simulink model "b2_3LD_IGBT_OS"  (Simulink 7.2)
settings: Solver=ode3  SolverMode=SingleTasking  StartTime=0.0  StopTime=0.2  FixedStep=10e-6  MaxStep=1e-5  RelTol=1e-4  AbsTol=1e-4

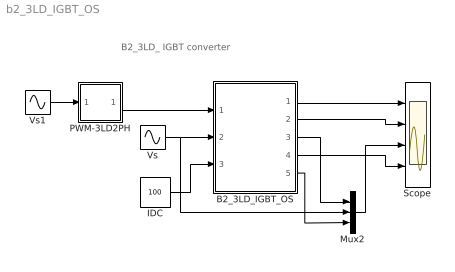
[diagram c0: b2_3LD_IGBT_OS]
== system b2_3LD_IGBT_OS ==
  note: B2_3LD_ IGBT converter
  B2_3LD_IGBT_OS : Subsystem  mask(B2-3-Level NPC IGBT Converter){LS=2e-3, C=20e-3, VC0=200, RL=10e5}
      mask prompts: LS "Source Inductance"; C "Load Cap"; VC0 "Initial Cap Voltage"; RL "Load Resistance"
      mask help: Input Vector u: u[0]= IGBT1.gate u[1]= IGBT2.gate u[2]= IGBT3.gate u[3]= IGBT4.gate u[4]= IGBT5.gate u[5]= IGBT6.gate u[6]= IGBT7.gate u[7]= IGBT8.gate u[8]= V1.V u[9]= IDC.i Output Vector y: y[0]= T1.I y[1]= D1.I y[2]= T1.V y[3]= T2.I y[4]= D2.I y[5]= T2.V y[6]= LS1.I y[7]= DC.V y[8]= Va.V Parameter Vector p: p[0]= Ls.L p[1]= C1.C p[2]= C1.vC0 p[3]= R1.r You can pause the simulation during running, change the Parameters you want and continue the Simulation
  IDC : Constant  Value=100
  Mux2 : Mux  Inputs=3
  PWM-3LD2PH : Subsystem  mask(PWM-3LD_3PH){FT=900, PHT=0, A=0.5, O1=0.5, O2=-0.5, DT=1e-6}
      mask prompts: FT "Frequency of Trian Sig."; PHT "Phase Angle of Trian. Sig."; A "Amplitude of Trian. Sig."; O1 "Offset of 1st Trian"; O2 "Offset of 2nd Trian."; DT "Dead Time"
      mask help: Pulse Width Modulation for 2 Legs of 3 Level Neutral point clamped Converter
  Scope : Scope  NumInputPorts=4
  Vs : Sin  Amplitude=230*sqrt(2)  Frequency=50*2*pi  SampleTime=0
  Vs1 : Sin  Amplitude=0.74  Frequency=50*2*pi  Phase=-pi/6  SampleTime=0
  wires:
  IDC/1 -> B2_3LD_IGBT_OS/3(iDC)
  B2_3LD_IGBT_OS/1(iT1,iD1,vT1) -> Scope/1
  B2_3LD_IGBT_OS/2(iT2,iD2,vT2) -> Scope/2
  B2_3LD_IGBT_OS/4(vDC12) -> Scope/4
  Vs/1 -> Mux2/2, B2_3LD_IGBT_OS/2(vS)
  Vs1/1 -> PWM-3LD2PH/1(In1)
  B2_3LD_IGBT_OS/3(iLs) -> Mux2/1
  Mux2/1 -> Scope/3
  B2_3LD_IGBT_OS/5(va) -> Mux2/3
  PWM-3LD2PH/1(Out1) -> B2_3LD_IGBT_OS/1(SWs)

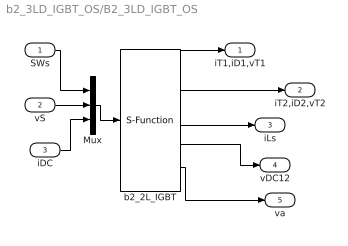
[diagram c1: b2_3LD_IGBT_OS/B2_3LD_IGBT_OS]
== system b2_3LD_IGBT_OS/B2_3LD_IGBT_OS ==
  SWs : Inport  OutDataType=sfix(16)  OutScaling=2^0
  vS : Inport  Port=2  OutDataType=sfix(16)  OutScaling=2^0
  iDC : Inport  Port=3  OutDataType=sfix(16)  OutScaling=2^0
  Mux : Mux  Inputs="[8  1  1]"
  b2_2L_IGBT : S-Function  FunctionName=s_b2_3LD_IGBT_OS  Parameters="[ LS  C  VC0 RL]"  EnableBusSupport=off
  iT1,iD1,vT1 : Outport  OutDataType=sfix(16)  OutScaling=2^0
  iT2,iD2,vT2 : Outport  Port=2  OutDataType=sfix(16)  OutScaling=2^0
  iLs : Outport  Port=3  OutDataType=sfix(16)  OutScaling=2^0
  vDC12 : Outport  Port=4  OutDataType=sfix(16)  OutScaling=2^0
  va : Outport  Port=5  OutDataType=sfix(16)  OutScaling=2^0
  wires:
  b2_2L_IGBT/4 -> vDC12/1
  Mux/1 -> b2_2L_IGBT/1
  iDC/1 -> Mux/3
  b2_2L_IGBT/3 -> iLs/1
  b2_2L_IGBT/2 -> iT2,iD2,vT2/1
  b2_2L_IGBT/1 -> iT1,iD1,vT1/1
  vS/1 -> Mux/2
  SWs/1 -> Mux/1
  b2_2L_IGBT/5 -> va/1

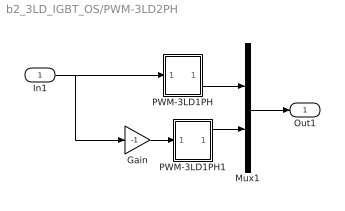
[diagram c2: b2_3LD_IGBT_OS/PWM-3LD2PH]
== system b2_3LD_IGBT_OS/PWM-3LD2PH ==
  In1 : Inport  OutDataType=sfix(16)  OutScaling=2^0
  Gain : Gain  Gain=-1  ParameterDataType=sfix(16)  ParameterScaling=2^0  OutDataType=sfix(16)  OutScaling=2^0
  Mux1 : Mux  Inputs=2
  PWM-3LD1PH : Subsystem  mask(PWM-3LD1PH){FT=FT, PHT=PHT, A=A, O1=O1, O2=O2, DT=DT}
      mask prompts: FT "Frequency of Trian Sig."; PHT "Phase Angle of Trian. Sig."; A "Amplitude of Trian. Sig."; O1 "Offset of 1st Trian"; O2 "Offset of 2nd Trian."; DT "Dead Time"
      mask help: Pulse Width Modulation for 1 Phase 3 Level Floating Capacitor Converter
  PWM-3LD1PH1 : Subsystem  mask(PWM-3LD1PH){FT=FT, PHT=PHT, A=A, O1=O1, O2=O2, DT=DT}
      mask prompts: FT "Frequency of Trian Sig."; PHT "Phase Angle of Trian. Sig."; A "Amplitude of Trian. Sig."; O1 "Offset of 1st Trian"; O2 "Offset of 2nd Trian."; DT "Dead Time"
      mask help: Pulse Width Modulation for 1 Phase 3 Level Floating Capacitor Converter
  Out1 : Outport
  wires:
  PWM-3LD1PH1/1(Out1) -> Mux1/2
  PWM-3LD1PH/1(Out1) -> Mux1/1
  In1/1 -> Gain/1, PWM-3LD1PH/1(In1)
  Gain/1 -> PWM-3LD1PH1/1(In1)
  Mux1/1 -> Out1/1

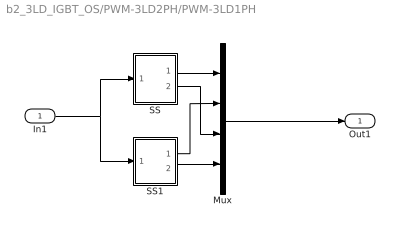
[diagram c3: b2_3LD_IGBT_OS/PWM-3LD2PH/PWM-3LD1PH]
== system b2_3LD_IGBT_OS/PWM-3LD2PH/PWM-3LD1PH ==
  In1 : Inport  OutDataType=sfix(16)  OutScaling=2^0
  Mux : Mux
  SS : Subsystem
  SS1 : Subsystem
  Out1 : Outport
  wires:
  In1/1 -> SS1/1(I1), SS/1(I1)
  SS1/1(O1) -> Mux/2
  SS/2(O2) -> Mux/3
  Mux/1 -> Out1/1
  SS/1(O1) -> Mux/1
  SS1/2(O2) -> Mux/4

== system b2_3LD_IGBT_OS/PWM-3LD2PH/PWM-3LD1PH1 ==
  In1 : Inport  OutDataType=sfix(16)  OutScaling=2^0
  Mux : Mux
  SS : Subsystem
  SS1 : Subsystem
  Out1 : Outport
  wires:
  SS1/2(O2) -> Mux/4
  SS/1(O1) -> Mux/1
  Mux/1 -> Out1/1
  SS/2(O2) -> Mux/3
  SS1/1(O1) -> Mux/2
  In1/1 -> SS/1(I1), SS1/1(I1)

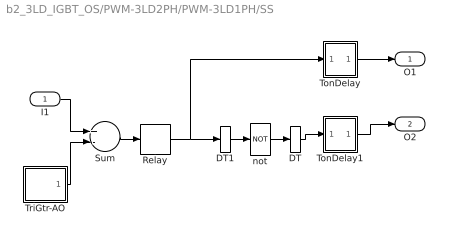
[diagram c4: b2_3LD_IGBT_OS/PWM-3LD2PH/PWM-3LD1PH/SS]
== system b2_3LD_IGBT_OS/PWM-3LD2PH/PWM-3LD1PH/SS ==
  I1 : Inport  OutDataType=sfix(16)  OutScaling=2^0
  DT : DataTypeConversion
  DT1 : DataTypeConversion
  Relay : Relay  OutDataType=sfix(16)  OutScaling=2^0
  Sum : Sum  Inputs=+-  OutDataType=sfix(16)  OutScaling=2^0
  TonDelay : Subsystem  mask(TonDelay){DT=DT}
      mask prompts: DT "Dead Time"
      mask help: Turn on dead time to protect against short circuit of the converter leg
  TonDelay1 : Subsystem  mask(TonDelay){DT=DT}
      mask prompts: DT "Dead Time"
      mask help: Turn on dead time to protect against short circuit of the converter leg
  TriGtr-AO : Subsystem  mask(TriGtr-AO){A=A, O=O1, T=1/FT, Td=PHT/FT/180}
      mask prompts: A "Amplitude"; O "Offset"; T "Period Time"; Td "Time Delay"
      mask help: Triangular Wave Generator with variable time delay, variable amplitude and offset
  not : Logic  Operator=NOT  Inputs=1
  O1 : Outport  InitialOutput=0
  O2 : Outport  Port=2  InitialOutput=0
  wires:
  TonDelay/1(s1d) -> O1/1
  Relay/1 -> TonDelay/1(s1), DT1/1
  TonDelay1/1(s1d) -> O2/1
  not/1 -> DT/1
  Sum/1 -> Relay/1
  TriGtr-AO/1(Out1) -> Sum/2
  I1/1 -> Sum/1
  DT/1 -> TonDelay1/1(s1)
  DT1/1 -> not/1

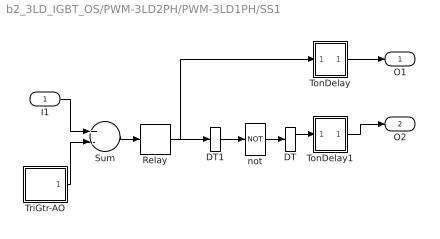
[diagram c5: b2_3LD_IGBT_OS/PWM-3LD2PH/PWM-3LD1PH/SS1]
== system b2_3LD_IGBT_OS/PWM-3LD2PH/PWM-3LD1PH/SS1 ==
  I1 : Inport  OutDataType=sfix(16)  OutScaling=2^0
  DT : DataTypeConversion
  DT1 : DataTypeConversion
  Relay : Relay  OutDataType=sfix(16)  OutScaling=2^0
  Sum : Sum  Inputs=+-  OutDataType=sfix(16)  OutScaling=2^0
  TonDelay : Subsystem  mask(TonDelay){DT=DT}
      mask prompts: DT "Dead Time"
      mask help: Turn on dead time to protect against short circuit of the converter leg
  TonDelay1 : Subsystem  mask(TonDelay){DT=DT}
      mask prompts: DT "Dead Time"
      mask help: Turn on dead time to protect against short circuit of the converter leg
  TriGtr-AO : Subsystem  mask(TriGtr-AO){A=A, O=O2, T=1/FT, Td=PHT/FT/180}
      mask prompts: A "Amplitude"; O "Offset"; T "Period Time"; Td "Time Delay"
      mask help: Triangular Wave Generator with variable time delay, variable amplitude and offset
  not : Logic  Operator=NOT  Inputs=1
  O1 : Outport  InitialOutput=0
  O2 : Outport  Port=2  InitialOutput=0
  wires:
  TonDelay/1(s1d) -> O1/1
  Relay/1 -> TonDelay/1(s1), DT1/1
  TonDelay1/1(s1d) -> O2/1
  not/1 -> DT/1
  Sum/1 -> Relay/1
  TriGtr-AO/1(Out1) -> Sum/2
  I1/1 -> Sum/1
  DT/1 -> TonDelay1/1(s1)
  DT1/1 -> not/1

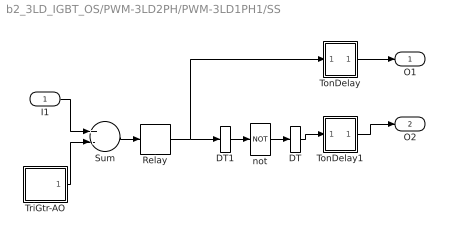
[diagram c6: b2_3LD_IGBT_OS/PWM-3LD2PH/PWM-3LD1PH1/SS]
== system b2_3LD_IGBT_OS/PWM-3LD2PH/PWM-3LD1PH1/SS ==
  I1 : Inport  OutDataType=sfix(16)  OutScaling=2^0
  DT : DataTypeConversion
  DT1 : DataTypeConversion
  Relay : Relay  OutDataType=sfix(16)  OutScaling=2^0
  Sum : Sum  Inputs=+-  OutDataType=sfix(16)  OutScaling=2^0
  TonDelay : Subsystem  mask(TonDelay){DT=DT}
      mask prompts: DT "Dead Time"
      mask help: Turn on dead time to protect against short circuit of the converter leg
  TonDelay1 : Subsystem  mask(TonDelay){DT=DT}
      mask prompts: DT "Dead Time"
      mask help: Turn on dead time to protect against short circuit of the converter leg
  TriGtr-AO : Subsystem  mask(TriGtr-AO){A=A, O=O1, T=1/FT, Td=PHT/FT/180}
      mask prompts: A "Amplitude"; O "Offset"; T "Period Time"; Td "Time Delay"
      mask help: Triangular Wave Generator with variable time delay, variable amplitude and offset
  not : Logic  Operator=NOT  Inputs=1
  O1 : Outport  InitialOutput=0
  O2 : Outport  Port=2  InitialOutput=0
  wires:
  DT1/1 -> not/1
  DT/1 -> TonDelay1/1(s1)
  I1/1 -> Sum/1
  TriGtr-AO/1(Out1) -> Sum/2
  Sum/1 -> Relay/1
  not/1 -> DT/1
  TonDelay1/1(s1d) -> O2/1
  Relay/1 -> DT1/1, TonDelay/1(s1)
  TonDelay/1(s1d) -> O1/1

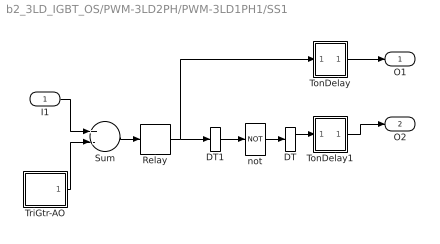
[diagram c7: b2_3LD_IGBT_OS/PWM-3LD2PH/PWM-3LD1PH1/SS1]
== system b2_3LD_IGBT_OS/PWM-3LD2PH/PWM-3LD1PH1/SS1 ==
  I1 : Inport  OutDataType=sfix(16)  OutScaling=2^0
  DT : DataTypeConversion
  DT1 : DataTypeConversion
  Relay : Relay  OutDataType=sfix(16)  OutScaling=2^0
  Sum : Sum  Inputs=+-  OutDataType=sfix(16)  OutScaling=2^0
  TonDelay : Subsystem  mask(TonDelay){DT=DT}
      mask prompts: DT "Dead Time"
      mask help: Turn on dead time to protect against short circuit of the converter leg
  TonDelay1 : Subsystem  mask(TonDelay){DT=DT}
      mask prompts: DT "Dead Time"
      mask help: Turn on dead time to protect against short circuit of the converter leg
  TriGtr-AO : Subsystem  mask(TriGtr-AO){A=A, O=O2, T=1/FT, Td=PHT/FT/180}
      mask prompts: A "Amplitude"; O "Offset"; T "Period Time"; Td "Time Delay"
      mask help: Triangular Wave Generator with variable time delay, variable amplitude and offset
  not : Logic  Operator=NOT  Inputs=1
  O1 : Outport  InitialOutput=0
  O2 : Outport  Port=2  InitialOutput=0
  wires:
  DT1/1 -> not/1
  DT/1 -> TonDelay1/1(s1)
  I1/1 -> Sum/1
  TriGtr-AO/1(Out1) -> Sum/2
  Sum/1 -> Relay/1
  not/1 -> DT/1
  TonDelay1/1(s1d) -> O2/1
  Relay/1 -> DT1/1, TonDelay/1(s1)
  TonDelay/1(s1d) -> O1/1

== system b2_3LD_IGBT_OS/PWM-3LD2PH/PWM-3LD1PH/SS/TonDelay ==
  s1 : Inport  Orientation=down  OutDataType=sfix(16)  OutScaling=2^0
  Int : Integrator  ExternalReset=falling
  Rel1 : Relay  OnSwitchValue=DT  OutDataType=sfix(16)  OutScaling=2^0
  s1d : Outport  InitialOutput=0
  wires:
  Rel1/1 -> s1d/1
  s1/1 -> Int/1, Int/2
  Int/1 -> Rel1/1

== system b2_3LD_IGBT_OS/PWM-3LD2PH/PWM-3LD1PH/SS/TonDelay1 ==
  s1 : Inport  Orientation=down  OutDataType=sfix(16)  OutScaling=2^0
  Int : Integrator  ExternalReset=falling
  Rel1 : Relay  OnSwitchValue=DT  OutDataType=sfix(16)  OutScaling=2^0
  s1d : Outport  InitialOutput=0
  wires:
  Rel1/1 -> s1d/1
  s1/1 -> Int/1, Int/2
  Int/1 -> Rel1/1

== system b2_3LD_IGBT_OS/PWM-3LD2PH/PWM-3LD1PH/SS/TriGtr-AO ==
  Ampl. : Gain  Gain=A  ParameterDataType=sfix(16)  ParameterScaling=2^0  OutDataType=sfix(16)  OutScaling=2^0
  Offset : Constant  Value=O  OutDataType=sfix(16)  OutScaling=2^0
  Sum : Sum  OutDataType=sfix(16)  OutScaling=2^0
  TriGtr : Subsystem  mask(TriGtr){T=1/FT, Td=PHT/FT/180}
      mask prompts: T "Period Time"; Td "Time Delay"
      mask help: Triangular Wave Generator with variable time delay
  Out1 : Outport
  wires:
  Sum/1 -> Out1/1
  Ampl./1 -> Sum/1
  TriGtr/1(O) -> Ampl./1
  Offset/1 -> Sum/2

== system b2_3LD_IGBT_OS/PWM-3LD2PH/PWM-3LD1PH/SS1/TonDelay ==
  s1 : Inport  Orientation=down  OutDataType=sfix(16)  OutScaling=2^0
  Int : Integrator  ExternalReset=falling
  Rel1 : Relay  OnSwitchValue=DT  OutDataType=sfix(16)  OutScaling=2^0
  s1d : Outport  InitialOutput=0
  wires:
  Rel1/1 -> s1d/1
  s1/1 -> Int/1, Int/2
  Int/1 -> Rel1/1

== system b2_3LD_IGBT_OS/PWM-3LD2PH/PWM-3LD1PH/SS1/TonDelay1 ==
  s1 : Inport  Orientation=down  OutDataType=sfix(16)  OutScaling=2^0
  Int : Integrator  ExternalReset=falling
  Rel1 : Relay  OnSwitchValue=DT  OutDataType=sfix(16)  OutScaling=2^0
  s1d : Outport  InitialOutput=0
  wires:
  Rel1/1 -> s1d/1
  s1/1 -> Int/1, Int/2
  Int/1 -> Rel1/1

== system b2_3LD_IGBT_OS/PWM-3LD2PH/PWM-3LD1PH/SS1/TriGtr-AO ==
  Ampl. : Gain  Gain=A  ParameterDataType=sfix(16)  ParameterScaling=2^0  OutDataType=sfix(16)  OutScaling=2^0
  Offset : Constant  Value=O  OutDataType=sfix(16)  OutScaling=2^0
  Sum : Sum  OutDataType=sfix(16)  OutScaling=2^0
  TriGtr1 : Subsystem  mask(TriGtr){T=1/FT, Td=PHT/FT/180}
      mask prompts: T "Period Time"; Td "Time Delay"
      mask help: Triangular Wave Generator with variable time delay
  Out1 : Outport
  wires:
  Offset/1 -> Sum/2
  TriGtr1/1(O) -> Ampl./1
  Ampl./1 -> Sum/1
  Sum/1 -> Out1/1

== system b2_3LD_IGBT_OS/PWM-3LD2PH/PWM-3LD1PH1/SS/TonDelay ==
  s1 : Inport  Orientation=down  OutDataType=sfix(16)  OutScaling=2^0
  Int : Integrator  ExternalReset=falling
  Rel1 : Relay  OnSwitchValue=DT  OutDataType=sfix(16)  OutScaling=2^0
  s1d : Outport  InitialOutput=0
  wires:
  Int/1 -> Rel1/1
  s1/1 -> Int/2, Int/1
  Rel1/1 -> s1d/1

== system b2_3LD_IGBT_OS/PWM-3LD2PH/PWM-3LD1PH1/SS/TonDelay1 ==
  s1 : Inport  Orientation=down  OutDataType=sfix(16)  OutScaling=2^0
  Int : Integrator  ExternalReset=falling
  Rel1 : Relay  OnSwitchValue=DT  OutDataType=sfix(16)  OutScaling=2^0
  s1d : Outport  InitialOutput=0
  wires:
  Int/1 -> Rel1/1
  s1/1 -> Int/2, Int/1
  Rel1/1 -> s1d/1

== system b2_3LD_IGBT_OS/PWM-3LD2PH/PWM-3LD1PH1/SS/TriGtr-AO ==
  Ampl. : Gain  Gain=A  ParameterDataType=sfix(16)  ParameterScaling=2^0  OutDataType=sfix(16)  OutScaling=2^0
  Offset : Constant  Value=O  OutDataType=sfix(16)  OutScaling=2^0
  Sum : Sum  OutDataType=sfix(16)  OutScaling=2^0
  TriGtr : Subsystem  mask(TriGtr){T=1/FT, Td=PHT/FT/180}
      mask prompts: T "Period Time"; Td "Time Delay"
      mask help: Triangular Wave Generator with variable time delay
  Out1 : Outport
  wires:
  Offset/1 -> Sum/2
  TriGtr/1(O) -> Ampl./1
  Ampl./1 -> Sum/1
  Sum/1 -> Out1/1

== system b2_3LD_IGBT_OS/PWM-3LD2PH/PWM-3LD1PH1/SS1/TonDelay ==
  s1 : Inport  Orientation=down  OutDataType=sfix(16)  OutScaling=2^0
  Int : Integrator  ExternalReset=falling
  Rel1 : Relay  OnSwitchValue=DT  OutDataType=sfix(16)  OutScaling=2^0
  s1d : Outport  InitialOutput=0
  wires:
  Int/1 -> Rel1/1
  s1/1 -> Int/2, Int/1
  Rel1/1 -> s1d/1

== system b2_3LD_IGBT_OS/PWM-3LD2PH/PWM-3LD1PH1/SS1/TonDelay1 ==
  s1 : Inport  Orientation=down  OutDataType=sfix(16)  OutScaling=2^0
  Int : Integrator  ExternalReset=falling
  Rel1 : Relay  OnSwitchValue=DT  OutDataType=sfix(16)  OutScaling=2^0
  s1d : Outport  InitialOutput=0
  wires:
  Int/1 -> Rel1/1
  s1/1 -> Int/2, Int/1
  Rel1/1 -> s1d/1

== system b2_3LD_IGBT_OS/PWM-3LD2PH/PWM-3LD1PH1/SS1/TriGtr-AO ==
  Ampl. : Gain  Gain=A  ParameterDataType=sfix(16)  ParameterScaling=2^0  OutDataType=sfix(16)  OutScaling=2^0
  Offset : Constant  Value=O  OutDataType=sfix(16)  OutScaling=2^0
  Sum : Sum  OutDataType=sfix(16)  OutScaling=2^0
  TriGtr : Subsystem  mask(TriGtr){T=1/FT, Td=PHT/FT/180}
      mask prompts: T "Period Time"; Td "Time Delay"
      mask help: Triangular Wave Generator with variable time delay
  Out1 : Outport
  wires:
  Sum/1 -> Out1/1
  Ampl./1 -> Sum/1
  TriGtr/1(O) -> Ampl./1
  Offset/1 -> Sum/2

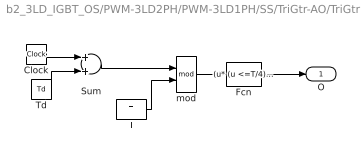
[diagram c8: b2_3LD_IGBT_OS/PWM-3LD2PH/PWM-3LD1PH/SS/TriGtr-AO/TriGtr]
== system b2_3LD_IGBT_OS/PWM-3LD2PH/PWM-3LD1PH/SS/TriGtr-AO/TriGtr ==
  Clock : Clock
  Fcn : Fcn  Expr="(u* (u <=T/4) * 4/T)   +  (  (u > T/4) && ( u <=3*T/4) )* ( 1 - (u-T/4) *4/T )   +  ( (u > 3*T/4)&& (u<=T)) * ( ((u -3*T/4)* 4/T )-1 )"
  Sum : Sum
  T : Constant  Value=T
  Td : Constant  Value=Td
  mod : Math  Operator=mod
  O : Outport  InitialOutput=0
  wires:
  mod/1 -> Fcn/1
  Fcn/1 -> O/1
  Clock/1 -> Sum/1
  T/1 -> mod/2
  Sum/1 -> mod/1
  Td/1 -> Sum/2

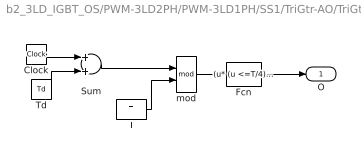
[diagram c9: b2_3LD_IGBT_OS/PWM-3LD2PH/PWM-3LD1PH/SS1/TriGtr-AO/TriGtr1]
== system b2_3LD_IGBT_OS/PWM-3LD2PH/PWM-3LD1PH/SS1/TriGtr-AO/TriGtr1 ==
  Clock : Clock
  Fcn : Fcn  Expr="(u* (u <=T/4) * 4/T)   +  (  (u > T/4) && ( u <=3*T/4) )* ( 1 - (u-T/4) *4/T )   +  ( (u > 3*T/4)&& (u<=T)) * ( ((u -3*T/4)* 4/T )-1 )"
  Sum : Sum
  T : Constant  Value=T
  Td : Constant  Value=Td
  mod : Math  Operator=mod
  O : Outport  InitialOutput=0
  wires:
  Td/1 -> Sum/2
  Sum/1 -> mod/1
  T/1 -> mod/2
  Clock/1 -> Sum/1
  Fcn/1 -> O/1
  mod/1 -> Fcn/1

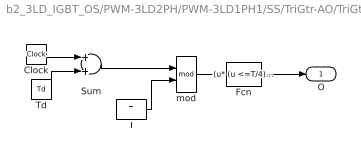
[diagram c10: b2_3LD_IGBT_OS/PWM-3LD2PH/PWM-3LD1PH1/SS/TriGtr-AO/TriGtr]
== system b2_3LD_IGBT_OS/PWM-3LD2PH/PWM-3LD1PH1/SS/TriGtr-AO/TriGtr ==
  Clock : Clock
  Fcn : Fcn  Expr="(u* (u <=T/4) * 4/T)   +  (  (u > T/4) && ( u <=3*T/4) )* ( 1 - (u-T/4) *4/T )   +  ( (u > 3*T/4)&& (u<=T)) * ( ((u -3*T/4)* 4/T )-1 )"
  Sum : Sum
  T : Constant  Value=T
  Td : Constant  Value=Td
  mod : Math  Operator=mod
  O : Outport  InitialOutput=0
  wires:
  Td/1 -> Sum/2
  Sum/1 -> mod/1
  T/1 -> mod/2
  Clock/1 -> Sum/1
  Fcn/1 -> O/1
  mod/1 -> Fcn/1

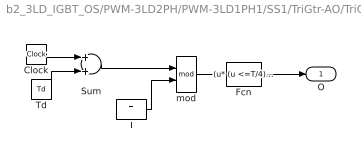
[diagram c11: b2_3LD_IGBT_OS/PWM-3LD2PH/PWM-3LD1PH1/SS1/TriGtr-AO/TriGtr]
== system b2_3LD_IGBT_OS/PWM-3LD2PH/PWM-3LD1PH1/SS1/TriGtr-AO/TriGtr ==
  Clock : Clock
  Fcn : Fcn  Expr="(u* (u <=T/4) * 4/T)   +  (  (u > T/4) && ( u <=3*T/4) )* ( 1 - (u-T/4) *4/T )   +  ( (u > 3*T/4)&& (u<=T)) * ( ((u -3*T/4)* 4/T )-1 )"
  Sum : Sum
  T : Constant  Value=T
  Td : Constant  Value=Td
  mod : Math  Operator=mod
  O : Outport  InitialOutput=0
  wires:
  Td/1 -> Sum/2
  Sum/1 -> mod/1
  T/1 -> mod/2
  Clock/1 -> Sum/1
  Fcn/1 -> O/1
  mod/1 -> Fcn/1
